FUNCTION_BLOCK Example15_DOdisplacement //4x3 flyways 1 xbot - DO set on displacement
VAR_INPUT
	Execute : BOOL;
END_VAR
VAR_OUTPUT
	Done : BOOL;
END_VAR
VAR_IN_OUT
	PM_Controller : PMControllerType;	// the planar motor controller to use
END_VAR
VAR
	PMC_XYMotion1 : PMC_XYMotion;
	DoID_array5 : ARRAY[0..4] OF USINT;
	xbotID_array5 : ARRAY[0..4] OF USINT;
	type_array5 : ARRAY[0..4] OF USINT;
	mode_array5 : ARRAY[0..4] OF USINT;
	threshold_array5 : ARRAY[0..4] OF REAL;
	xfactor_array5 : ARRAY[0..4] OF REAL;
	yfactor_array5 : ARRAY[0..4] OF REAL;
	PMC_ConfigDO2Disp1 : PMC_ConfigDO2Disp;
	PMC_XYMotion2 : PMC_XYMotion;
	first_read : BOOL;
	PMC_ReadDigitalSignalFromPMC1 : PMC_ReadDigitalSignalFromPMC;
	DI_ID_array22 : ARRAY[0..21] OF USINT;
	Rst_DO_ID_array22 : ARRAY[0..21] OF USINT;
	PMC_ConfigDI2Reset1 : PMC_ConfigDI2Reset;
	PMC_SendDigitalSignalToPMC1 : PMC_SendDigitalSignalToPMC;
	Delay1 : Delay;
	PMC_SendDigitalSignalToPMC2 : PMC_SendDigitalSignalToPMC;
	Delay2 : Delay;
	second_read : BOOL;
	PMC_ReadDigitalSignalFromPMC2 : PMC_ReadDigitalSignalFromPMC;
END_VAR

//4x3 flyways 1 xbot - DO set on displacement

//move xbot 1 to 60,60
PMC_XYMotion1(Execute := Execute,cmdLB := 1,XbotID := 1,Mode := 0,Type_ := 0,PosX := 0.06,PosY := 0.06,EndVel := 0,MaxVel := 1,MaxAcc := 10,PM_Controller := PM_Controller);

//config DO1 to set on a x > 500 
DoID_array5[0] := 1;
xbotID_array5[0] := 1;
type_array5[0] := 0;
mode_array5[0] := 0;
threshold_array5[0] := 0.500;
PMC_ConfigDO2Disp1(Execute := PMC_XYMotion1.Done,nDO := 1,DoID := DoID_array5,XbotID := xbotID_array5,Type_ := type_array5,Mode := mode_array5,Threshold := threshold_array5,XFactor := xfactor_array5,YFactor := yfactor_array5,PM_Controller := PM_Controller);

//move xbot 1 to 900,60
PMC_XYMotion2(Execute := PMC_ConfigDO2Disp1.Done,cmdLB := 3,XbotID := 1,Mode := 0,Type_ := 0,PosX := 0.9,PosY := 0.06,EndVel := 0,MaxVel := 1,MaxAcc := 10,PM_Controller := PM_Controller);

//read DO 1 
PMC_ReadDigitalSignalFromPMC1(Enable := PMC_XYMotion2.Done,DiID := 1,PM_Controller := PM_Controller);
//only record the output of the first read once
IF(PMC_ReadDigitalSignalFromPMC1.Valid = TRUE AND PMC_ConfigDI2Reset1.Done = FALSE)THEN
	first_read := PMC_ReadDigitalSignalFromPMC1.Level;
END_IF;

//setup DI 1 as reset for DO 1
DI_ID_array22[0] := 1;
Rst_DO_ID_array22[0] := 1;
PMC_ConfigDI2Reset1(Execute := PMC_ReadDigitalSignalFromPMC1.Valid,nDI := 1,DiID := DI_ID_array22,RstDoID := Rst_DO_ID_array22,PM_Controller := PM_Controller);

//set DI 1 to 0
PMC_SendDigitalSignalToPMC1(Enable := PMC_ConfigDI2Reset1.Done,DoID := 1,Level := FALSE,PM_Controller := PM_Controller);

Delay1(Execute := PMC_SendDigitalSignalToPMC1.Valid,Cycles := 1);

//set DI 1 to 1
PMC_SendDigitalSignalToPMC2(Enable := Delay1.Done,DoID := 1,Level := TRUE,PM_Controller := PM_Controller);

Delay2(Execute := PMC_SendDigitalSignalToPMC2.Valid,Cycles := 1);

//read DO1
PMC_ReadDigitalSignalFromPMC2(Enable := Delay2.Done,DiID := 1,Level => second_read,PM_Controller := PM_Controller);

Done := PMC_ReadDigitalSignalFromPMC2.Valid;

END_FUNCTION_BLOCK
